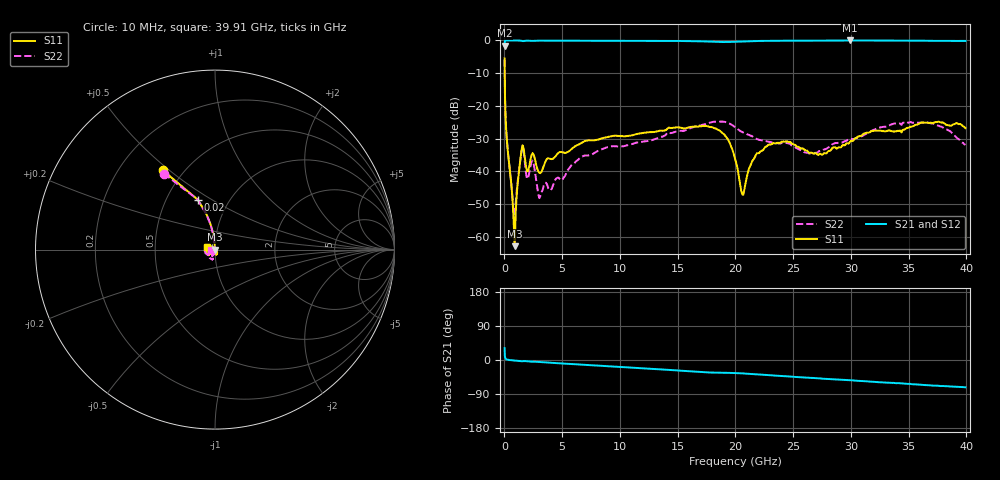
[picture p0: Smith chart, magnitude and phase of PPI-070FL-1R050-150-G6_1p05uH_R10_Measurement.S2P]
! Data measured by Modelithics Inc.  support@modelithics.com  813-866-6335  Tampa FL USA June 2025
! PPI-070FL-1R050-150-G6_1p05uH measured on 10-mil thick RO4350B board, mounted in 2-port shunt configuration on a 50-ohm transmission line
# Hz S MA R 50
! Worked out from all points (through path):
!   429 points, 10 MHz to 39.91 GHz, reference 50 ohm
!   highest |S21| = 0.00 dB at 29.91 GHz (marker M1); lowest = -1.6 dB at 10 MHz (marker M2)
!   group delay of S21, straight-line fit = 5.08 ps
!   lowest |S11| = -62.9 dB at 882.5 MHz (marker M3), VSWR 1.00, Z = 49.9 - j0.0313 ohm
!   |S11| at or under -10 dB: 18.75 MHz to end of sweep
!   |S22| runs from -53.2 to -5.8 dB; largest |S21 - S12| = 0.026
!   S11 on the Smith chart (normalised r, x): 10 MHz: 0.38, +0.47; 20 MHz: 0.72, +0.44; 39.91 GHz: 0.92, +0.03
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1e7  0.5307 123.4  0.8335 31.4  0.8333 31.4  0.5101 124.0
2e7  0.2938 108.9  0.9467 17.1  0.9465 17.1  0.2955 109.1
7e7  0.08956 96.9  0.9929 5.0  0.9927 5.0  0.08963 97.5
2e8  0.03075 93.9  0.9981 1.4  0.9979 1.4  0.03082 95.3
6.883552e8  0.003876 99.2  0.9989 -1.0  0.9987 -1.0  0.004076 114.5
8.825328e8  0.0007186 -154.2  0.9988 -1.5  0.9985 -1.5  0.002198 -170.5
1.562154e9  0.02506 -145.5  0.9787 -3.3  0.9785 -3.3  0.02355 -163.3
1.950509e9  0.009945 -168.7  0.9912 -3.4  0.991 -3.4  0.007677 176.1
2.533042e9  0.01797 -172.8  0.9844 -4.4  0.9841 -4.4  0.01288 165.0
3.115575e9  0.009379 -154.7  0.9934 -5.6  0.9932 -5.5  0.004247 -154.6
6.70786e9  0.0274 -134.4  0.9891 -12.3  0.9887 -12.3  0.01679 -95.0
1.340699e10  0.0416 -141.5  0.9854 -24.6  0.9851 -24.7  0.03306 -111.2
1.816434e10  0.04565 -172.8  0.9532 -33.3  0.9529 -33.6  0.05722 -164.8
2.000902e10  0.01455 120.1  0.9575 -34.4  0.9573 -34.5  0.04651 155.1
2.059156e10  0.004419 51.1  0.9667 -35.2  0.9664 -35.5  0.03996 151.7
2.165953e10  0.01616 -45.6  0.9803 -37.3  0.9801 -37.4  0.03233 152.3
2.28246e10  0.02529 -61.9  0.9888 -39.7  0.9884 -39.7  0.02835 162.1
2.670815e10  0.01879 -97.1  0.9926 -47.3  0.9922 -47.3  0.01879 -166.1
2.991208e10  0.0281 -167.5  0.9995 -53.4  0.999 -53.7  0.03071 -123.6
3.331019e10  0.04212 -178.8  0.9945 -59.9  0.9941 -60.1  0.05001 -105.4
3.709665e10  0.05484 169.2  0.9861 -67.5  0.9858 -67.1  0.05382 -130.1
3.991223e10  0.04588 160.3  0.9838 -72.1  0.9834 -71.6  0.02536 -169.9
